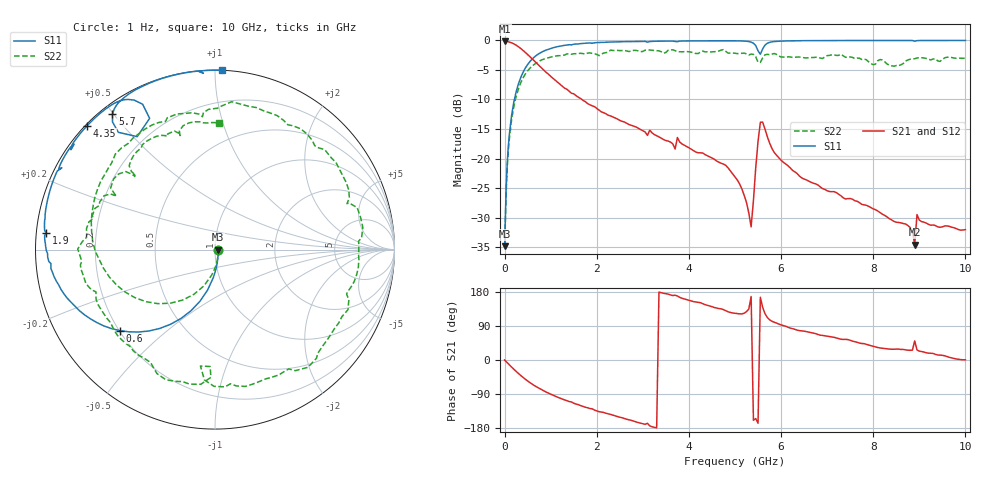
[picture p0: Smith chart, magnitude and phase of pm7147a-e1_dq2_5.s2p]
# GHz S DB R 50
! S-Parameters data
! Freq  dbS11  angS11  dbS21  angS21  dbS12  angS12  dbS22  angS22
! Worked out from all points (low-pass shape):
!   279 points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, 1 Hz to 10 GHz, reference 50 ohm
!   highest |S21| = -0.16 dB at 398.1 Hz (marker M1); lowest = -34.6 dB at 8.9 GHz (marker M2)
!   |S21| within 3 dB of the highest: start of sweep to 602.4 MHz
!   lowest |S11| = -34.8 dB at 398.1 Hz (marker M3), VSWR 1.04, Z = 51.8 - j6.37e-05 ohm
!   |S11| at or under -10 dB: start of sweep to 212.8 MHz
!   |S22| runs from -34.8 to -1.6 dB; largest |S21 - S12| = 3.3e-14
!   S11 on the Smith chart (normalised r, x): 1 Hz: 1.04, -0.00; 600 MHz: 0.20, -0.35; 1.9 GHz: 0.03, +0.05; 4.35 GHz: 0.00, +0.41; 5.7 GHz: 0.03, +0.50; 10 GHz: 0.00, +1.04
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1e-09  -34.84 -0.0  -0.16 -0.0  -0.16 -0.0  -34.84 -0.0
3.981e-07  -34.84 -0.0  -0.16 -0.0  -0.16 -0.0  -34.84 -0.0
0.05011872  -21.90 -81.8  -0.19 -6.2  -0.19 -6.2  -22.60 -83.0
0.15  -12.77 -100.4  -0.40 -18.4  -0.40 -18.4  -13.52 -107.0
0.35  -6.28 -120.8  -1.36 -40.9  -1.36 -40.9  -7.17 -136.5
0.6  -3.14 -139.6  -3.14 -63.8  -3.14 -63.8  -4.32 -165.4
1.05  -1.24 -161.8  -6.41 -92.8  -6.41 -92.8  -2.73 156.2
1.7  -0.50 178.9  -10.13 -122.5  -10.13 -122.5  -2.22 113.8
1.9  -0.48 174.3  -11.07 -128.8  -11.07 -128.8  -2.19 102.4
2.55  -0.22 162.0  -13.70 -152.3  -13.70 -152.3  -1.72 68.2
3.35  -0.13 149.5  -16.33 179.1  -16.33 179.1  -1.77 24.0
4.35  -0.07 135.9  -19.33 146.0  -19.33 146.0  -1.94 -27.9
5.05  -0.07 126.4  -23.63 122.6  -23.63 122.6  -2.23 -68.4
5.35  -0.29 120.1  -31.58 167.4  -31.58 167.4  -2.31 -85.8
5.55  -2.34 124.6  -13.86 165.7  -13.86 165.7  -3.72 -92.4
5.7  -0.49 127.2  -16.25 112.4  -16.25 112.4  -2.35 -100.7
6.7  -0.03 113.0  -24.17 71.0  -24.17 71.0  -2.89 -152.2
7.3  -0.02 107.4  -26.31 54.8  -26.31 54.8  -2.33 179.7
8.35  -0.01 98.9  -30.17 28.8  -30.17 28.8  -4.18 137.8
8.9  -0.13 93.8  -34.57 50.5  -34.57 50.5  -3.10 126.0
8.95  -0.03 95.2  -29.48 26.5  -29.48 26.5  -2.97 124.7
10  -0.00 87.7  -32.04 0.5  -32.04 0.5  -3.01 88.0
